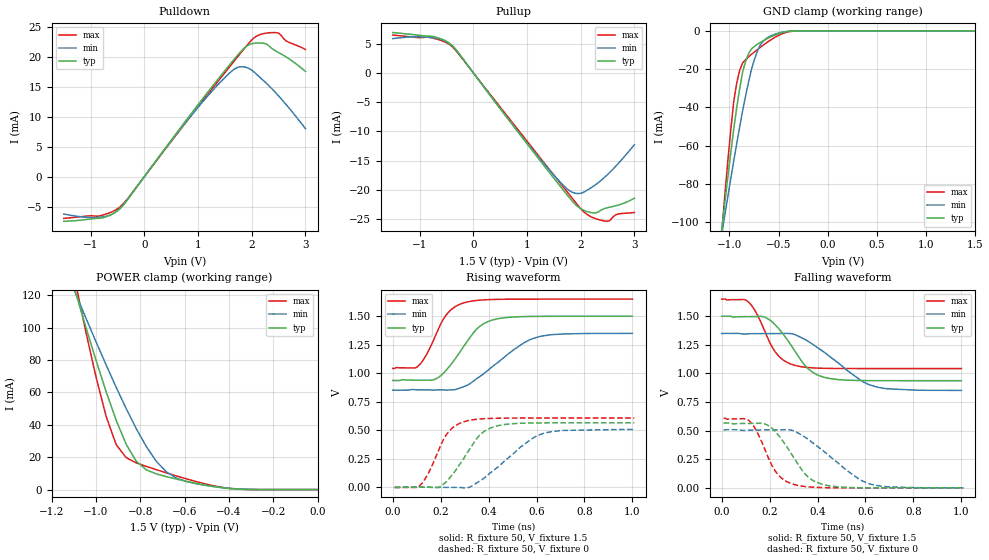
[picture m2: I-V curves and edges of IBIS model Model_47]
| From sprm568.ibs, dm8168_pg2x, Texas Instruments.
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| Model based on original model for BSHTLTCSCDVGPBFZ
|   Sub model FAST_5MA_10PER_1P5
[model]   Model_47
|[Description]  [1.5V-3-STATE-X-FAST:5MA, IND, 10%]
|   Fast slew rate (SR[1:0] = "10"), 1.60 * RExt = 0.625 * Iout
|   (I[2:0] = "000"), 5mA nominal with Rext = 50R, ,Industrial
|   temperature range (-40C to 125C, 25C nominal),10% power supply
|   tolerance
|[Input Load]
|[Output Drive] FAST:5MA
|Voltage   1.5V
|Mode   3-STATE
Model_type   3-state
Polarity   Non-Inverting
Enable   Active-Low
Cref =  15.0000pF
Rref =  100.0000M
Vref =  0V
Vmeas =  0.75
C_comp   1.5249p   1.4275p   1.6205p
[Model Spec]
[Temperature Range]   25   125   -40
[Voltage Range]   1.5   1.35   1.65
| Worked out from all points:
|   slope of the pulldown table from 0 to 0.225 V, typ, clamps not added: 81.7 ohm
|   slope of the pullup table from 0 to 0.225 V, typ, clamps not added: 81.7 ohm
|   GND clamp passes 1 mA (typ) near -0.47 V on its own axis
|   POWER clamp passes 1 mA (typ) near -0.42 V on its own axis
|   rising waveform, R_fixture 50, V_fixture 1.5: 20-80 % time 118ps typ, 186ps min, 89.2ps max; typ from 0.937 V to 1.5 V
|   rising waveform, R_fixture 50, V_fixture 0: 20-80 % time 112ps typ, 175ps min, 84.9ps max; typ from 0 V to 0.566 V
|   falling waveform, R_fixture 50, V_fixture 1.5: 20-80 % time 117ps typ, 190ps min, 88.3ps max; typ from 1.5 V to 0.937 V
|   falling waveform, R_fixture 50, V_fixture 0: 20-80 % time 112ps typ, 184ps min, 84.8ps max; typ from 0.566 V to 0 V
[POWER_clamp]
-1.5V     321.6mA    260.6mA    415.8mA
-1.091V   121.1mA    120.8mA    126.6mA
-1.076V   114.1mA    115.8mA    116.8mA
-1V       79.88mA    91.3mA     69.56mA
-954.5mV  60.58mA    77.05mA    45.34mA
-909.1mV  42.84mA    63.2mA     27.8mA
-818.2mV  17.47mA    37.6mA     16.51mA
-772.7mV  12.19mA    26.53mA    14.33mA
-681.8mV  7.985mA    10.89mA    10.33mA
-590.9mV  5.092mA    4.952mA    6.596mA
-363.6mV  298.9uA    465.6uA    298.1uA
0V        1.518nA    23.05nA    396.5pA
[Pulldown]
-1.5V     -7.45mA    -6.24mA    -6.96mA
-863.6mV  -6.95mA    -6.794mA   -6.6mA
-500mV    -5.682mA   -5.687mA   -5.359mA
-318.2mV  -3.897mA   -3.877mA   -3.74mA
1V        12mA       11.57mA    11.65mA
1.455V    17.18mA    16.12mA    16.83mA
1.727V    20.16mA    18.19mA    19.88mA
2V        22.16mA    17.76mA    22.81mA
2.318V    21.82mA    15.17mA    23.99mA
2.5V      20.69mA    13.46mA    23.94mA
2.636V    19.99mA    12.06mA    22.66mA
3V        17.55mA    8mA        21.21mA
[Pullup]
-1.5V     6.87mA     5.84mA     6.44mA
-818.2mV  6.271mA    6.054mA    6.043mA
-409.1mV  4.8mA      4.74mA     4.606mA
1.227V    -14.81mA   -14.54mA   -14.31mA
1.682V    -20.1mA    -19.29mA   -19.58mA
1.864V    -22.13mA   -20.48mA   -21.67mA
2V        -23.22mA   -20.59mA   -23.2mA
2.182V    -23.86mA   -19.71mA   -24.55mA
2.409V    -23.31mA   -18.15mA   -25.25mA
2.545V    -22.95mA   -16.97mA   -25.21mA
2.682V    -22.64mA   -15.67mA   -24.17mA
3V        -21.43mA   -12.28mA   -23.87mA
[GND_clamp]
-1.5V     -310mA     -250.5mA   -402.4mA
-1.076V   -103.5mA   -106.1mA   -105.2mA
-1.045V   -89.74mA   -96.32mA   -85.93mA
-954.5mV  -51.19mA   -67.85mA   -36.85mA
-924.2mV  -40.06mA   -58.84mA   -27.27mA
-863.6mV  -21.23mA   -41.55mA   -16.73mA
-833.3mV  -15.79mA   -33.74mA   -15.03mA
-772.7mV  -9.342mA   -19.74mA   -12.19mA
-712.1mV  -6.927mA   -10.35mA   -9.702mA
-621.2mV  -4.26mA    -3.894mA   -6.224mA
-409.1mV  -336.9uA   -288.9uA   -618.6uA
1.5V      1.518nA    2.298uA    269.6pA
[Ramp]
dV/dt_f   0.450808/0.17888912n   0.398752/0.27111023n   0.486/0.14046315n
dV/dt_r 0.45446208/0.17056215n 0.40963016/0.25116841n 0.48679116/0.1357847n
R_load = 50
[Rising Waveform]
R_fixture = 50
V_fixture = 1.5
V_fixture_min = 1.35
V_fixture_max = 1.65
0s        937.3mV    852.6mV    1.043V
105.6ps   940.2mV    855mV      1.063V
140.5ps   939.5mV    854.5mV    1.162V
191.7ps   965.5mV    854.3mV    1.393V
239.6ps   1.069V     853.8mV    1.55V
293.2ps   1.226V     880.5mV    1.615V
351.7ps   1.39V      955.2mV    1.639V
402.3ps   1.457V     1.035V     1.646V
609.3ps   1.499V     1.321V     1.65V
1ns       1.5V       1.35V      1.65V
[Rising Waveform]
R_fixture = 50
V_fixture = 0
V_fixture_min = 0
V_fixture_max = 0
8.21ps    0V         0V         0V
110.6ps   3.367mV    3.036mV    11.98mV
149.1ps   2.216mV    2.358mV    125.7mV
198ps     8.44mV     2.027mV    358.5mV
242.1ps   95.68mV    0V         507.9mV
296.8ps   255.4mV    -3.716mV   575.7mV
358.7ps   448.4mV    50.78mV    598.9mV
408.3ps   521mV      129.9mV    604.8mV
622.8ps   565.5mV    469.5mV    608.3mV
1.008ns   566.4mV    508.1mV    608.4mV
[Falling Waveform]
R_fixture = 50
V_fixture = 1.5
V_fixture_min = 1.35
V_fixture_max = 1.65
0s        1.499V     1.349V     1.649V
109.9ps   1.496V     1.346V     1.628V
141.9ps   1.497V     1.347V     1.539V
178.1ps   1.494V     1.348V     1.378V
225.3ps   1.421V     1.348V     1.183V
303.5ps   1.202V     1.34V      1.072V
353.4ps   1.056V     1.29V      1.053V
407.5ps   979.7mV    1.215V     1.046V
615.6ps   937.3mV    901.5mV    1.042V
1ns       936.6mV    851.7mV    1.042V
[Falling Waveform]
R_fixture = 50
V_fixture = 0
V_fixture_min = 0
V_fixture_max = 0
8.21ps    565.8mV    507.4mV    607.8mV
115.6ps   562.6mV    504.7mV    584.7mV
149.7ps   564.1mV    505.2mV    479.4mV
200.2ps   537mV      506.1mV    236.9mV
241.8ps   446.8mV    507.2mV    100.7mV
291.1ps   296.9mV    503.8mV    36.3mV
344.8ps   129.8mV    446.7mV    12.01mV
386.6ps   57.67mV    382.9mV    5.471mV
615.7ps   0V         36.35mV    0V
1.008ns   0V         0V         0V
